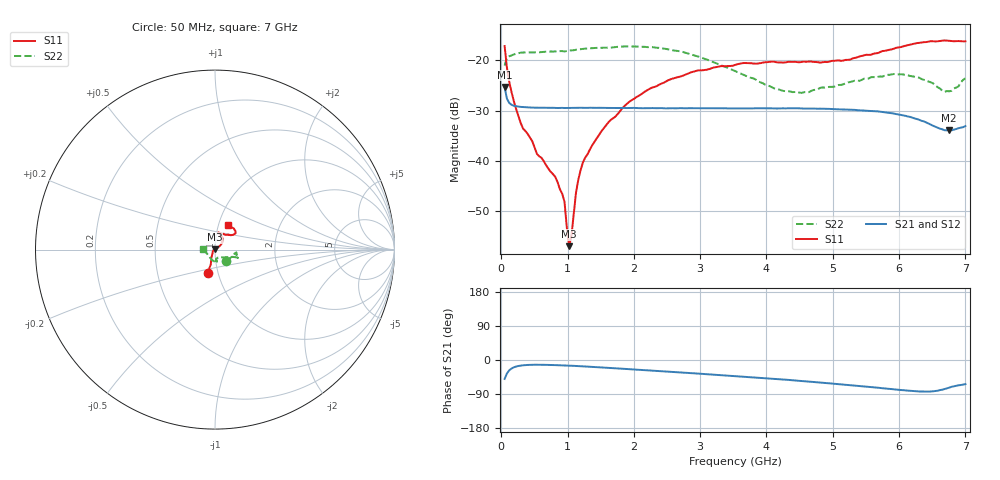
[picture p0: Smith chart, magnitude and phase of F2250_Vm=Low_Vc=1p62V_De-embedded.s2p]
! Integrated Device Technology
! Corporate Headquarters
! 6024 Silver Creek Valley Road
! San Jose, CA 95138  USA
! Phone:  1-408-284-8200
! Toll Free:  1-800-223-1366
! Webpage:  http://www.idt.com/
! Timing and RF Division
! 515 Groton Road, Suite 102
! Westford, MA 01886-6024
! Device:  F2250
! Description: Voltage Variable RF Attenuator
! Frequency:  50.0 -  6000.00 MHz
! Package:  3x3 mm Thin QFN Plastic Package: 16 pin
! Ports:  2 RF, 3 DC
!  Pin  1  = GND
!  Pin  2  = NC
!  Pin  3  = RF1  = Port 1
!  Pin  4  = NC
!  Pin  5  = GND
!  Pin  6  = GND
!  Pin  7  = GND
!  Pin  8  = GND
!  Pin  9  = NC
!  Pin 10  = RF2  = Port 2
!  Pin 11  = NC
!  Pin 12  = GND
!  Pin 13  = GND
!  Pin 14  = VCNTRL
!  Pin 15  = VDD
!  Pin 16  = VMODE
! Vcntrl:  1.620 Volts
! Vmode:  +0.000 Volts
! Vdd:  +3.30  Volts
! Current:  1.190 mA
! Data:  The device was measured on a the F2250 evaluation board which has
!  individual transmission lines to the RF pins.  Data was collected
!  using a calibrated network analyzer.  The evaluation board was
!  de-embedded using a TRL calibration technique.
!  The reference plane is the edge of the package pin.
! Misc:  SN 10
!  Action Tracker AT0258
! Date Measured:  2014-11-26
! Date:  2015-10-15  MJV
! Note:
!  Integrated Device Technology supplies this data as a sample of measured
!  data at the package pin for this product.  Your particular data for this
!  product may vary.
!  Data was taken at 25 degrees C.
!  Integrated Device Technology reserves the right to change this data at anytime.
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# GHz S dB R 50
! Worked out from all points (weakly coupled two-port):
!   201 points, 50 MHz to 7 GHz, reference 50 ohm
!   highest |S21| = -25.30 dB at 50 MHz (marker M1); lowest = -34.0 dB at 6.757 GHz (marker M2)
!   lowest |S11| = -57.0 dB at 1.023 GHz (marker M3), VSWR 1.00, Z = 49.9 + j0.119 ohm
!   |S11| at or under -10 dB: start of sweep to end of sweep
!   |S22| runs from -26.5 to -17.2 dB; largest |S21 - S12| = 0.00019
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0.05  -17.16 -107.5  -25.30 -49.9  -25.30 -49.9  -21.04 -45.8
0.1195  -24.23 -109.8  -28.47 -27.3  -28.48 -27.3  -19.20 -13.3
0.29325  -32.50 -123.5  -29.27 -14.7  -29.27 -14.7  -18.48 -8.6
0.5365  -38.61 -149.7  -29.43 -12.5  -29.42 -12.5  -18.42 -8.7
0.8145  -43.21 175.4  -29.47 -13.5  -29.46 -13.5  -18.23 -12.3
0.91875  -46.56 156.4  -29.47 -14.2  -29.48 -14.2  -18.16 -13.9
0.9535  -48.16 173.9  -29.49 -14.4  -29.50 -14.4  -18.25 -13.9
1.023  -56.99 122.7  -29.47 -14.9  -29.47 -14.9  -18.06 -14.2
1.05775  -54.95 81.6  -29.46 -15.2  -29.48 -15.2  -18.04 -14.4
1.12725  -46.29 42.3  -29.45 -15.7  -29.45 -15.8  -17.90 -15.4
1.2315  -40.31 33.8  -29.46 -16.7  -29.47 -16.7  -17.73 -16.7
1.6485  -31.89 37.9  -29.48 -21.1  -29.49 -21.1  -17.47 -18.4
1.9265  -28.30 38.7  -29.49 -24.2  -29.49 -24.1  -17.25 -19.3
2.37825  -24.87 45.5  -29.52 -29.2  -29.52 -29.2  -17.52 -20.0
2.93425  -22.11 58.7  -29.54 -35.5  -29.57 -35.4  -19.09 -21.6
3.525  -20.93 71.6  -29.58 -42.5  -29.58 -42.5  -22.14 -33.4
4.25475  -20.45 77.4  -29.56 -51.5  -29.59 -51.5  -26.10 -59.8
4.7065  -20.32 71.9  -29.61 -58.0  -29.60 -58.0  -25.92 -78.0
5.85325  -17.90 39.9  -30.47 -76.2  -30.47 -76.3  -22.89 -83.6
6.305  -16.53 40.2  -31.85 -83.0  -31.92 -83.1  -23.47 -92.5
6.75675  -16.11 50.8  -33.95 -72.9  -34.02 -72.8  -26.17 -145.7
7  -16.21 62.9  -33.09 -63.7  -33.15 -63.4  -23.57 179.0
